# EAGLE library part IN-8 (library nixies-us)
IN-8: medium numeric frontview nixie tube
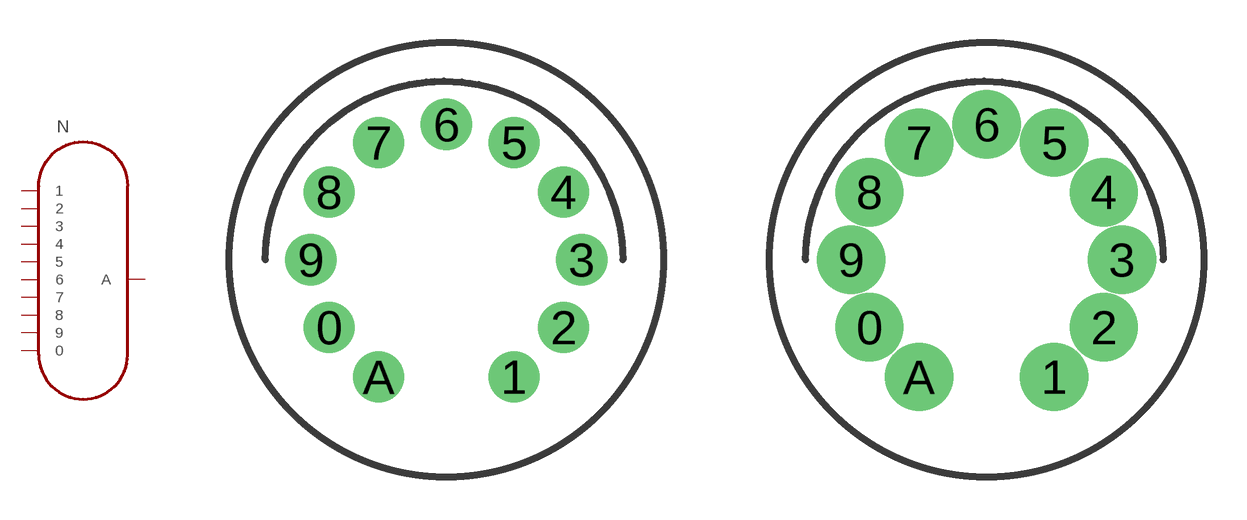
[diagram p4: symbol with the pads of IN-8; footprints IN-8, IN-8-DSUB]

Designator prefix N

## IN-8  [IN-8]
0  0
1  1
2  2
3  3
4  4
5  5
6  6
7  7
8  8
9  9
A  A

## IN-8DSUB  [IN-8-DSUB]
Pads as for IN-8

## Footprint IN-8 (pad centres in mm)
May be used with socket: 11-pin- Russian
drill 1.2: 0 -4.114,-2.375; 1 2.375,-4.114; 2 4.114,-2.375; 3 4.75,0; 4 4.114,2.375; 5 2.375,4.114; 6 0,4.75; 7 -2.375,4.114; 8 -4.114,2.375; 9 -4.75,0; A -2.375,-4.114

## Footprint IN-8-DSUB (pad centres in mm)
May be used with socket: 11-pin- Russian
drill 1.6 pad 2.184: 0 -4.114,-2.375; 1 2.375,-4.114; 2 4.114,-2.375; 3 4.75,0; 4 4.114,2.375; 5 2.375,4.114; 6 0,4.75; 7 -2.375,4.114; 8 -4.114,2.375; 9 -4.75,0; A -2.375,-4.114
